|Texas Instruments Incorporated
| DDC2256 256-Channel, Current-Input Analog-To-Digital Converter
| Marketing part#   Digital Voltage Range   Package-type   #pins
| DDC2256   1.7V-1.9V   BGA   323
[IBIS Ver]   4.1
[File name]   ddc2256.ibs
[File Rev]   1.0
[Date]   1/22/2016
[Source]
| Texas Instruments Incorporated.
| Analog-eLab Design Center, HPA
| 12500 TI Blvd
| Dallas, TX -75243
[Notes]   Revision History:
| Rev 1.0: 1/22/2016
| - Initial version of the model
| - Model generated from simulations in SPECTRE.
| - Model matched to SPICE simulation
| - C_comp although listed in numerical order of value are
|   obtained from varying PVT conditions. For PVT conditions for
|   each specific value refer the buffer description under
|   respective [Model]. IBIS model user is responsible for using
|   appropriate C_comp to simulate for Signal Integrity.
|* EXCEPTION:   *
|* - For clk model,there is leakage in power clamp/ground clamp IV   *
|*   tables due to resistors R2,R8 connected to pad.   *
|* - For sdout model,pullup and pulldown IV tables are not passing   *
|*   through zero due to resistors R3,R4,R5 and R6 connected to pad.   *
|* - For lvds model,pullup and pulldown IV tables are not passing   *
|*   through zero due to driver switch arrangement   *
[Disclaimer]
| This model is designed as an aid for customers of Texas Instruments.
| TI and its licensors and suppliers make no warranties, either expressed
| or implied, with respect to this  model, including the warranties of
| merchantability or fitness for a particular purpose. The model is
| provided solely on an "as is" basis. The entire risk as to its quality
| and performance is with the customer.
[Copyright]
(C) Copyright 2016 Texas Instruments Incorporated.All rights reserved.
|   DDC2256ZZF
[Component]   DDC2256ZZF
[Manufacturer]   TI
[Package]   |323 BGA  -  ZZF Package
|   typ   min   max
R_pkg   0.01   0.008   0.012
L_pkg   0.1nH   0.08nH   0.12nH
C_pkg   0.1pF   0.08pF   0.12pF
[Pin]  signal_name   model_name   R_pin   L_pin   C_pin
A1   IN3   nc   NA   NA   NA
A2   IN2   nc   NA   NA   NA
A3   IN1   nc   NA   NA   NA
A4   IN20   nc   NA   NA   NA
A5   IN13   nc   NA   NA   NA
A6   IN11   nc   NA   NA   NA
A7   IN10   nc   NA   NA   NA
A8   QGND   gnd   NA   NA   NA
A9   IN4   nc   NA   NA   NA
A10   QGND   gnd   NA   NA   NA
A11   IN74   nc   NA   NA   NA
A12   IN75   nc   NA   NA   NA
A13   IN77   nc   NA   NA   NA
A14   IN84   nc   NA   NA   NA
A15   IN65   nc   NA   NA   NA
A16   IN66   nc   NA   NA   NA
A17   IN67   nc   NA   NA   NA
B1   IN6   nc   NA   NA   NA
B2   IN5   nc   NA   NA   NA
B3   IN130   nc   NA   NA   NA
B4   IN21   nc   NA   NA   NA
B5   IN14   nc   NA   NA   NA
B6   IN15   nc   NA   NA   NA
B7   IN19   nc   NA   NA   NA
B8   IN9   nc   NA   NA   NA
B9   IN68   nc   NA   NA   NA
B10   IN73   nc   NA   NA   NA
B11   IN83   nc   NA   NA   NA
B12   IN79   nc   NA   NA   NA
B13   IN78   nc   NA   NA   NA
B14   IN85   nc   NA   NA   NA
B15   IN194   nc   NA   NA   NA
B16   IN69   nc   NA   NA   NA
B17   IN70   nc   NA   NA   NA
C1   IN8   nc   NA   NA   NA
C2   IN7   nc   NA   NA   NA
C3   IN136   nc   NA   NA   NA
C4   IN133   nc   NA   NA   NA
C5   IN132   nc   NA   NA   NA
C6   IN131   nc   NA   NA   NA
C7   IN134   nc   NA   NA   NA
C8   IN129   nc   NA   NA   NA
C9   IN135   nc   NA   NA   NA
C10   IN193   nc   NA   NA   NA
C11   IN198   nc   NA   NA   NA
C12   IN195   nc   NA   NA   NA
C13   IN196   nc   NA   NA   NA
C14   IN197   nc   NA   NA   NA
C15   IN200   nc   NA   NA   NA
C16   IN71   nc   NA   NA   NA
C17   IN72   nc   NA   NA   NA
D1   IN16   nc   NA   NA   NA
D2   IN12   nc   NA   NA   NA
D3   IN140   nc   NA   NA   NA
D4   IN142   nc   NA   NA   NA
D5   IN141   nc   NA   NA   NA
D6   IN143   nc   NA   NA   NA
D7   IN139   nc   NA   NA   NA
D8   IN137   nc   NA   NA   NA
D9   IN199   nc   NA   NA   NA
D10   IN201   nc   NA   NA   NA
D11   IN203   nc   NA   NA   NA
D12   IN207   nc   NA   NA   NA
D13   IN205   nc   NA   NA   NA
D14   IN206   nc   NA   NA   NA
D15   IN204   nc   NA   NA   NA
D16   IN76   nc   NA   NA   NA
D17   IN80   nc   NA   NA   NA
E1   IN18   nc   NA   NA   NA
E2   IN17   nc   NA   NA   NA
E3   IN151   nc   NA   NA   NA
E4   IN22   nc   NA   NA   NA
E5   IN148   nc   NA   NA   NA
E6   IN147   nc   NA   NA   NA
E7   IN144   nc   NA   NA   NA
E8   IN145   nc   NA   NA   NA
E9   IN138   nc   NA   NA   NA
E10   IN202   nc   NA   NA   NA
E11   IN208   nc   NA   NA   NA
E12   IN211   nc   NA   NA   NA
E13   IN212   nc   NA   NA   NA
E14   IN86   nc   NA   NA   NA
E15   IN215   nc   NA   NA   NA
E16   IN81   nc   NA   NA   NA
E17   IN82   nc   NA   NA   NA
F1   IN24   nc   NA   NA   NA
F2   IN23   nc   NA   NA   NA
F3   IN30   nc   NA   NA   NA
F4   IN153   nc   NA   NA   NA
F5   IN26   nc   NA   NA   NA
F6   IN25   nc   NA   NA   NA
F7   IN149   nc   NA   NA   NA
F8   IN146   nc   NA   NA   NA
F9   IN209   nc   NA   NA   NA
F10   IN210   nc   NA   NA   NA
F11   IN213   nc   NA   NA   NA
F12   IN89   nc   NA   NA   NA
F13   IN90   nc   NA   NA   NA
F14   IN217   nc   NA   NA   NA
F15   IN94   nc   NA   NA   NA
F16   IN87   nc   NA   NA   NA
F17   IN88   nc   NA   NA   NA
G1   IN31   nc   NA   NA   NA
G2   IN29   nc   NA   NA   NA
G3   IN161   nc   NA   NA   NA
G4   IN32   nc   NA   NA   NA
G5   IN155   nc   NA   NA   NA
G6   IN28   nc   NA   NA   NA
G7   IN154   nc   NA   NA   NA
G8   IN152   nc   NA   NA   NA
G9   IN150   nc   NA   NA   NA
G10   IN214   nc   NA   NA   NA
G11   IN218   nc   NA   NA   NA
G12   IN92   nc   NA   NA   NA
G13   IN219   nc   NA   NA   NA
G14   IN96   nc   NA   NA   NA
G15   IN225   nc   NA   NA   NA
G16   IN93   nc   NA   NA   NA
G17   IN95   nc   NA   NA   NA
H1   IN37   nc   NA   NA   NA
H2   IN34   nc   NA   NA   NA
H3   IN38   nc   NA   NA   NA
H4   IN163   nc   NA   NA   NA
H5   IN159   nc   NA   NA   NA
H6   IN158   nc   NA   NA   NA
H7   IN157   nc   NA   NA   NA
H8   IN27   nc   NA   NA   NA
H9   IN216   nc   NA   NA   NA
H10   IN91   nc   NA   NA   NA
H11   IN221   nc   NA   NA   NA
H12   IN222   nc   NA   NA   NA
H13   IN223   nc   NA   NA   NA
H14   IN227   nc   NA   NA   NA
H15   IN102   nc   NA   NA   NA
H16   IN98   nc   NA   NA   NA
H17   IN101   nc   NA   NA   NA
J1   IN43   nc   NA   NA   NA
J2   IN39   nc   NA   NA   NA
J3   IN170   nc   NA   NA   NA
J4   IN168   nc   NA   NA   NA
J5   IN36   nc   NA   NA   NA
J6   IN35   nc   NA   NA   NA
J7   IN162   nc   NA   NA   NA
J8   IN160   nc   NA   NA   NA
J9   IN156   nc   NA   NA   NA
J10   IN220   nc   NA   NA   NA
J11   IN226   nc   NA   NA   NA
J12   IN99   nc   NA   NA   NA
J13   IN100   nc   NA   NA   NA
J14   IN232   nc   NA   NA   NA
J15   IN234   nc   NA   NA   NA
J16   IN103   nc   NA   NA   NA
J17   IN107   nc   NA   NA   NA
K1   IN47   nc   NA   NA   NA
K2   IN45   nc   NA   NA   NA
K3   IN175   nc   NA   NA   NA
K4   IN172   nc   NA   NA   NA
K5   IN167   nc   NA   NA   NA
K6   IN166   nc   NA   NA   NA
K7   IN165   nc   NA   NA   NA
K8   IN33   nc   NA   NA   NA
K9   IN224   nc   NA   NA   NA
K10   IN97   nc   NA   NA   NA
K11   IN229   nc   NA   NA   NA
K12   IN230   nc   NA   NA   NA
K13   IN231   nc   NA   NA   NA
K14   IN236   nc   NA   NA   NA
K15   IN239   nc   NA   NA   NA
K16   IN109   nc   NA   NA   NA
K17   IN111   nc   NA   NA   NA
L1   IN51   nc   NA   NA   NA
L2   IN48   nc   NA   NA   NA
L3   IN177   nc   NA   NA   NA
L4   IN173   nc   NA   NA   NA
L5   IN42   nc   NA   NA   NA
L6   IN171   nc   NA   NA   NA
L7   IN41   nc   NA   NA   NA
L8   IN40   nc   NA   NA   NA
L9   IN164   nc   NA   NA   NA
L10   IN228   nc   NA   NA   NA
L11   IN105   nc   NA   NA   NA
L12   IN235   nc   NA   NA   NA
L13   IN106   nc   NA   NA   NA
L14   IN237   nc   NA   NA   NA
L15   IN241   nc   NA   NA   NA
L16   IN112   nc   NA   NA   NA
L17   IN115   nc   NA   NA   NA
M1   IN53   nc   NA   NA   NA
M2   IN52   nc   NA   NA   NA
M3   IN184   nc   NA   NA   NA
M4   IN179   nc   NA   NA   NA
M5   IN178   nc   NA   NA   NA
M6   IN46   nc   NA   NA   NA
M7   IN44   nc   NA   NA   NA
M8   IN169   nc   NA   NA   NA
M9   IN104   nc   NA   NA   NA
M10   IN233   nc   NA   NA   NA
M11   IN108   nc   NA   NA   NA
M12   IN110   nc   NA   NA   NA
M13   IN242   nc   NA   NA   NA
M14   IN243   nc   NA   NA   NA
M15   IN248   nc   NA   NA   NA
M16   IN116   nc   NA   NA   NA
M17   IN117   nc   NA   NA   NA
N1   IN61   nc   NA   NA   NA
N2   IN57   nc   NA   NA   NA
N3   IN190   nc   NA   NA   NA
N4   IN191   nc   NA   NA   NA
N5   IN189   nc   NA   NA   NA
N6   IN185   nc   NA   NA   NA
N7   IN181   nc   NA   NA   NA
N8   IN180   nc   NA   NA   NA
N9   IN174   nc   NA   NA   NA
N10   IN238   nc   NA   NA   NA
N11   IN245   nc   NA   NA   NA
N12   IN249   nc   NA   NA   NA
N13   IN253   nc   NA   NA   NA
N14   IN255   nc   NA   NA   NA
N15   IN254   nc   NA   NA   NA
N16   IN121   nc   NA   NA   NA
N17   IN125   nc   NA   NA   NA
P1   IN64   nc   NA   NA   NA
P2   IN62   nc   NA   NA   NA
P3   IN58   nc   NA   NA   NA
P4   IN55   nc   NA   NA   NA
P5   IN50   nc   NA   NA   NA
P6   IN186   nc   NA   NA   NA
P7   IN183   nc   NA   NA   NA
P8   IN187   nc   NA   NA   NA
P9   IN244   nc   NA   NA   NA
P10   IN251   nc   NA   NA   NA
P11   IN247   nc   NA   NA   NA
P12   IN250   nc   NA   NA   NA
P13   IN114   nc   NA   NA   NA
P14   IN119   nc   NA   NA   NA
P15   IN122   nc   NA   NA   NA
P16   IN126   nc   NA   NA   NA
P17   IN128   nc   NA   NA   NA
R1   IN63   nc   NA   NA   NA
R2   IN182   nc   NA   NA   NA
R3   IN59   nc   NA   NA   NA
R4   IN56   nc   NA   NA   NA
R5   IN54   nc   NA   NA   NA
R6   IN192   nc   NA   NA   NA
R7   IN49   nc   NA   NA   NA
R8   IN176   nc   NA   NA   NA
R9   QGND   gnd   NA   NA   NA
R10   IN240   nc   NA   NA   NA
R11   IN113   nc   NA   NA   NA
R12   IN256   nc   NA   NA   NA
R13   IN118   nc   NA   NA   NA
R14   IN120   nc   NA   NA   NA
R15   IN123   nc   NA   NA   NA
R16   IN246   nc   NA   NA   NA
R17   IN127   nc   NA   NA   NA
T1   IN60   nc   NA   NA   NA
T2   IN188   nc   NA   NA   NA
T3   QGND   gnd   NA   NA   NA
T4   QGND   gnd   NA   NA   NA
T5   QGND   gnd   NA   NA   NA
T6   QGND   gnd   NA   NA   NA
T7   AGND   gnd   NA   NA   NA
T8   AGND   gnd   NA   NA   NA
T9   AGND   gnd   NA   NA   NA
T10   AGND   gnd   NA   NA   NA
T11   AGND   gnd   NA   NA   NA
T12   QGND   gnd   NA   NA   NA
T13   QGND   gnd   NA   NA   NA
T14   QGND   gnd   NA   NA   NA
T15   QGND   gnd   NA   NA   NA
T16   IN252   nc   NA   NA   NA
T17   IN124   nc   NA   NA   NA
U1   QGND   gnd   NA   NA   NA
U2   QGND   gnd   NA   NA   NA
U3   QGND   gnd   NA   NA   NA
U4   AGND   gnd   NA   NA   NA
U5   AGND   gnd   NA   NA   NA
U6   AGND   gnd   NA   NA   NA
U7   DVDD   power   NA   NA   NA
U8   DVDD   power   NA   NA   NA
U9   DGND   gnd   NA   NA   NA
U10   DGND   gnd   NA   NA   NA
U11   AGND   gnd   NA   NA   NA
U12   AGND   gnd   NA   NA   NA
U13   AGND   gnd   NA   NA   NA
U14   AGND   gnd   NA   NA   NA
U15   QGND   gnd   NA   NA   NA
U16   QGND   gnd   NA   NA   NA
U17   QGND   gnd   NA   NA   NA
V1   VREF_IN   nc   NA   NA   NA
V2   VREF_O   nc   NA   NA   NA
V3   AGND   gnd   NA   NA   NA
V4   AGND   gnd   NA   NA   NA
V5   CONV   nc   NA   NA   NA
V6   AGND   gnd   NA   NA   NA
V7   CLKM   clk   NA   NA   NA
V8   DCLKM   lvds   NA   NA   NA
V9   FCLKM   lvds   NA   NA   NA
V10   DOUTM   lvds   NA   NA   NA
V11   RESETZ   input   NA   NA   NA
V12   SENZ   input   NA   NA   NA
V13   AVEE   power   NA   NA   NA
V14   EN   nc   NA   NA   NA
V15   AGND   gnd   NA   NA   NA
V16   AGND   gnd   NA   NA   NA
V17   AGND   gnd   NA   NA   NA
W1   VRGND   gnd   NA   NA   NA
W2   VREF_C   nc   NA   NA   NA
W3   AVDD   power   NA   NA   NA
W4   AVDD   power   NA   NA   NA
W5   AVEE   power   NA   NA   NA
W6   AVEE   power   NA   NA   NA
W7   CLKP   clk   NA   NA   NA
W8   DCLKP   lvds   NA   NA   NA
W9   FCLKP   lvds   NA   NA   NA
W10   DOUTP   lvds   NA   NA   NA
W11   SCLK   input   NA   NA   NA
W12   SDIN   input   NA   NA   NA
W13   SDOUT   sdout   NA   NA   NA
W14   AGND   gnd   NA   NA   NA
W15   AVDD_18   power   NA   NA   NA
W16   AVDD_18   power   NA   NA   NA
W17   AVDD_18   power   NA   NA   NA
[Diff_pin]   inv_pin   vdiff   tdelay_typ   tdelay_min   tdelay_max
W7   V7   200mV   NA   NA   NA
W8   V8   NA   NA   NA   NA
W9   V9   NA   NA   NA   NA
W10   V10   NA   NA   NA   NA
| Models and submodels in the file (4): input (Input), sdout (Output), clk (Input), lvds (Output)
